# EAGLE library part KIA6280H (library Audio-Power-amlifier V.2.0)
22W BTL AUDIO POWER AMPLIFIER.
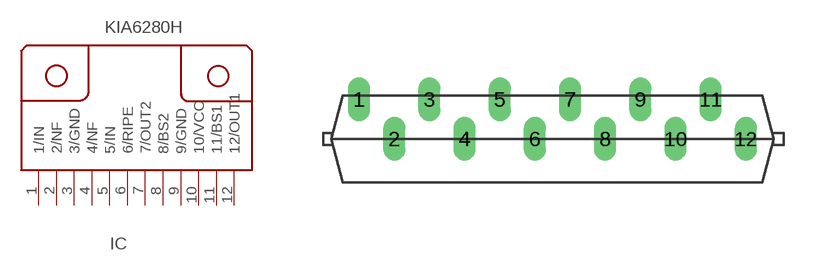
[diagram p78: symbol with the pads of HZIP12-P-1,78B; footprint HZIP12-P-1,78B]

Designator prefix IC

## KIA6280H  [HZIP12-P-1,78B]
1  1/IN  in
2  2/NF
3  3/GND  pwr
4  4/NF
5  5/IN  in
6  6/RIPE
7  7/OUT2  out
8  8/BS2
9  9/GND  pwr
10  10/VCC  pwr
11  11/BS1
12  12/OUT1  out

## Footprint HZIP12-P-1,78B (pad centres in mm)
drill 0.6 pad 1.016 long: 1 -9.779,2; 2 -8.001,0; 3 -6.223,2; 4 -4.445,0; 5 -2.667,2; 6 -0.889,0; 7 0.889,2; 8 2.667,0; 9 4.445,2; 10 6.223,0; 11 8.001,2; 12 9.779,0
